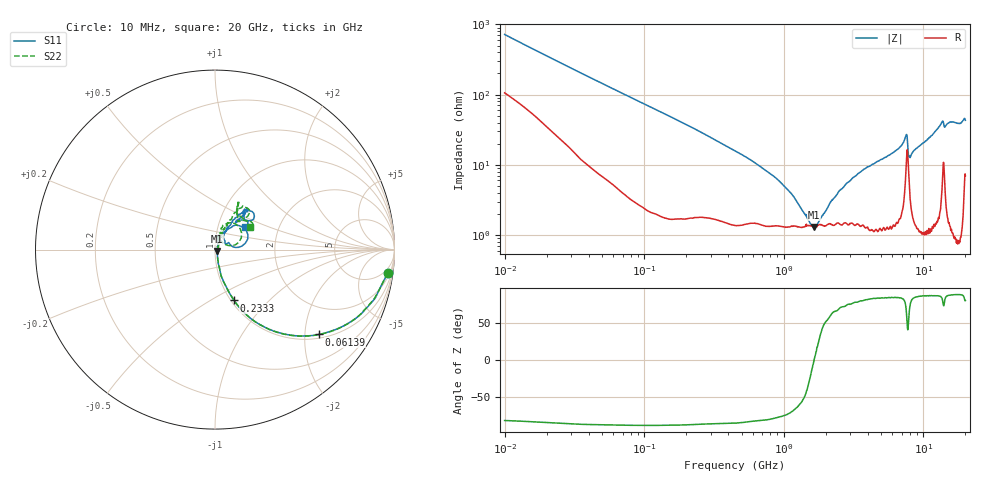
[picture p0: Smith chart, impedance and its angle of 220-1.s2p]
!Keysight Technologies,P5008B,MY61100088,A.16.20.02
!Date: Monday, May 27, 2024 17:28:56
!Correction: S11(C* 2-Port  )
!S21(C* 2-Port  )
!S12(C* 2-Port  )
!S22(C* 2-Port  )
!S2P File: Measurements: S11, S21, S12, S22:Log Frequency Sweep
# Hz S  dB  R 50
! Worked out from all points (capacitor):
!   1601 points, 10 MHz to 20 GHz, reference 50 ohm
!   read as one part in series: C = 22.5 pF near 10.39 MHz
!   lowest |Z| = 1.31 ohm at 1.644 GHz (marker M1)
!   series resonance near 1.648 GHz, so ESL is about 420 pH
!   S11 on the Smith chart (normalised r, x): 10 MHz: 3, -14; 61.39 MHz: 1.10, -2.36; 233.3 MHz: 1.03, -0.64; 20 GHz: 1.35, +0.36
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1e7  -0.24 -7.7  -17.38 73.8  -17.39 73.9  -0.26 -7.7
3.555162e7  -1.15 -25.7  -7.22 60.9  -7.23 60.9  -1.16 -25.8
6.139329e7  -2.52 -39.2  -3.96 48.3  -3.97 48.3  -2.53 -39.3
1.263918e8  -6.03 -58.3  -1.41 29.9  -1.43 29.9  -6.02 -58.3
2.332729e8  -10.39 -69.5  -0.56 17.4  -0.57 17.4  -10.41 -69.4
4.472136e8  -16.13 -76.6  -0.22 8.7  -0.24 8.7  -16.15 -76.7
9.206888e8  -23.96 -75.0  -0.12 3.0  -0.14 3.0  -24.06 -74.5
1.173095e9  -27.94 -69.4  -0.11 1.6  -0.13 1.6  -27.95 -67.2
1.589917e9  -36.18 -38.0  -0.10 -0.2  -0.12 -0.2  -34.65 -31.7
1.643677e9  -37.33 -33.1  -0.10 -0.4  -0.11 -0.4  -35.16 -25.3
1.959534e9  -37.26 27.8  -0.10 -1.4  -0.11 -1.4  -34.78 19.4
2.496738e9  -30.19 59.1  -0.10 -3.0  -0.12 -3.0  -29.51 52.5
3.810595e9  -24.62 78.3  -0.11 -6.3  -0.13 -6.3  -23.05 65.1
5.652411e9  -20.88 71.3  -0.12 -10.3  -0.14 -10.3  -20.61 71.8
7.410252e9  -14.96 49.8  -0.52 -16.6  -0.53 -16.6  -15.40 61.1
7.660815e9  -14.38 17.7  -1.32 -13.2  -1.33 -13.2  -15.88 24.1
8.148841e9  -23.41 34.6  -0.19 -12.2  -0.20 -12.2  -24.67 66.5
1.023592e10  -20.01 61.3  -0.10 -18.6  -0.12 -18.6  -19.65 65.9
1.341918e10  -11.30 52.6  -0.52 -27.4  -0.54 -27.3  -11.14 57.6
1.592205e10  -10.84 51.6  -0.41 -29.3  -0.42 -29.4  -10.68 62.9
1.827386e10  -14.23 53.3  -0.19 -33.9  -0.21 -33.9  -13.66 51.9
2e10  -13.52 36.6  -0.74 -36.5  -0.75 -36.6  -12.76 32.6
